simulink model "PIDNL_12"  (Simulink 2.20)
settings: Solver=VariableStepDiscrete  StartTime=0.0  StopTime=40.0  RelTol=1e-3  AbsTol=1e-6
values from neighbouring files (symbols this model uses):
  a = input('Inserisci il dato da graficare [1=PIDNL 2=PD 3=PID]: ')    [grp.m]    (also in grp1.m = input('Inserisci il dato da graficare [1..3]'))
undefined symbols (not defined in the file or in its folder): b, fnl, pidin
libraries: Puma x3, simulink x3

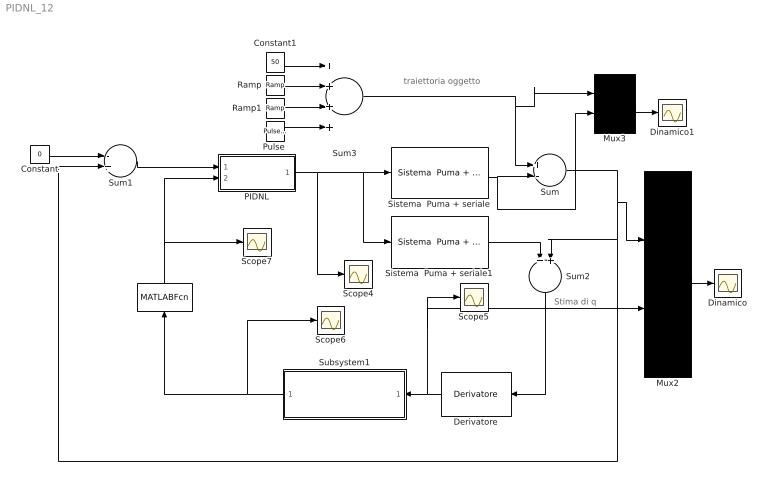
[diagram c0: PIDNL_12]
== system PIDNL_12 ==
  note: Stima di q
  note: traiettoria oggetto
  " " : MATLABFcn  Orientation=up  MATLABFcn=fnl(u(1))  OutputWidth=-1
  Constant : Constant  Value=0
  Constant1 : Constant  Value=50
  Derivatore : Puma/Derivatore  Orientation=left  Td=0.13  T=0.033  N=10
  Dinamico : Scope
  Dinamico1 : Scope
  Mux2 : Mux  Inputs=2
  Mux3 : Mux  Inputs=2
  PIDNL : Subsystem
  "Pulse " : simulink/Sources/Pulse Generator  period=30  duty=10  amplitude=-50  start=30
  Ramp : simulink/Sources/Ramp  slope=-50  start=10  X0=0
  Ramp1 : simulink/Sources/Ramp  slope=+50  start=25  X0=0
  Scope{4..7} (4 alike) : Scope
  Sistema  Puma + seriale : Puma/Sistema  Puma + seriale  Ts=.260
  Sistema  Puma + seriale1 : Puma/Sistema  Puma + seriale  Ts=.260
  Subsystem1 : Subsystem  Orientation=left  mask(Filtro di Butterworth){ordine=3, freq=0.1/16}
      mask prompts: ordine "Ordine del filtro"; freq "Parametro K per ricavare la Freq. di taglio Ft"
      mask help: Attenzione! Considerare il parametro Fc come la frequanza di campionamento del segnale di ingresso, per cui la frequanza di taglio diviene Ft=K*Fc;
      mask init:
      | [b,a]=butter(ordine,freq);
  Sum : Sum  Inputs=+-
  Sum1 : Sum  Inputs=-+
  Sum2 : Sum  Orientation=down  Inputs=++
  Sum3 : Sum  Inputs=++++
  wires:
  Sistema  Puma + seriale1/1 -> Sum2/1
  Mux2/1 -> Dinamico/1
  Sistema  Puma + seriale/1 -> Sum/2, Mux3/2
  Sum2/1 -> Derivatore/1
  Constant1/1 -> Sum3/1
  Sum1/1 -> PIDNL/1(In1)
  Constant/1 -> Sum1/1
  PIDNL/1(Out1) -> Sistema  Puma + seriale/1, Sistema  Puma + seriale1/1, Scope4/1
  Sum/1 -> Sum2/2, Sum1/2, Mux2/1
  Ramp/1 -> Sum3/2
  Ramp1/1 -> Sum3/3
  Mux3/1 -> Dinamico1/1
  Sum3/1 -> Sum/1, Mux3/1
  "Pulse "/1 -> Sum3/4
  Derivatore/1 -> Subsystem1/1(In1), Scope5/1, Mux2/2
  Subsystem1/1(Out1) -> " "/1, Scope6/1
  " "/1 -> PIDNL/2(In2), Scope7/1

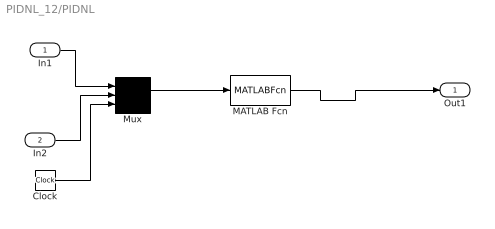
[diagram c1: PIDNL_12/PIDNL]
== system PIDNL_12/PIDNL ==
  In1 : Inport  Port=1  PortWidth=-1  SampleTime=-1
  In2 : Inport  Port=2  PortWidth=-1  SampleTime=-1
  Clock : Clock
  MATLAB Fcn : MATLABFcn  MATLABFcn=pidin(u(1),u(2),u(3))  OutputWidth=1
  Mux : Mux  Inputs=3
  Out1 : Outport  Port=1
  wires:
  MATLAB Fcn/1 -> Out1/1
  Mux/1 -> MATLAB Fcn/1
  In1/1 -> Mux/1
  In2/1 -> Mux/2
  Clock/1 -> Mux/3

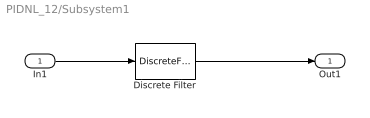
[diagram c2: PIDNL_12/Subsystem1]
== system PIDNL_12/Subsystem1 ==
  In1 : Inport  Port=1  PortWidth=-1  SampleTime=-1
  Discrete Filter : DiscreteFilter  Numerator=b  Denominator=a  SampleTime=.032
  Out1 : Outport  Port=1
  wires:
  In1/1 -> Discrete Filter/1
  Discrete Filter/1 -> Out1/1
